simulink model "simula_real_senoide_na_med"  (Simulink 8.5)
settings: Solver=ode45  StartTime=0.0  StopTime=tf  FixedStep=dt  RelTol=1e-9
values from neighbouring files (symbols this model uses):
  Areal = [zeros(n2,n2) eye(n2); -Pinv*R -Pinv*Q]    [mod_estados_real.m]
  Breal = [zeros(n2,1); Pinv*U]    [mod_estados_real.m]
  Creal = zeros(1,2*n2)    [mod_estados_real.m]
  denK = conv([1/3 1],[1 0.01])    [princi_JL_incerto_sem_prefilt_com_limit_ctrle.m]
  Dreal = 0    [mod_estados_real.m]
  numK = 3.5*0.1*[1 0.1]    [princi_JL_incerto_sem_prefilt_com_limit_ctrle.m]
  w0_med = wn    (= 10)    [princi_JL_incerto_sem_prefilt_com_limit_ctrle.m]

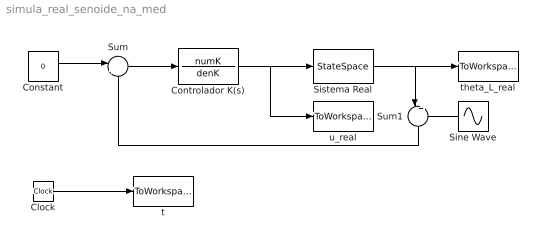
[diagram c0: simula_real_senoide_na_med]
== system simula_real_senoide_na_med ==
  Clock : Clock
  Constant : Constant  Value=0
  Controlador K(s) : TransferFcn  Numerator=numK  Denominator=denK
  Sine Wave : Sin  Frequency=w0_med  SampleTime=0
  Sistema Real : StateSpace  A=Areal  B=Breal  C=Creal  D=Dreal  X0=0
  Sum : Sum  Inputs=|+-
  Sum1 : Sum  Inputs=|++
  t : ToWorkspace  VariableName=t_real  SampleTime=-1
  theta_L_real : ToWorkspace  VariableName=theta_L_real  SampleTime=-1
  u_real : ToWorkspace  VariableName=u_real  SampleTime=-1
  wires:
  Sum/1 -> Controlador K(s)/1
  Constant/1 -> Sum/1
  Clock/1 -> t/1
  Controlador K(s)/1 -> u_real/1, Sistema Real/1
  Sine Wave/1 -> Sum1/2
  Sistema Real/1 -> Sum1/1, theta_L_real/1
  Sum1/1 -> Sum/2
